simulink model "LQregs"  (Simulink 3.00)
settings: Solver=ode45  StartTime=0.0  StopTime=100  RelTol=1e-3

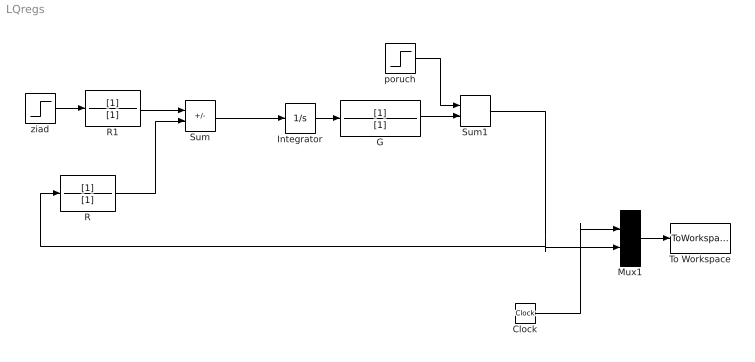
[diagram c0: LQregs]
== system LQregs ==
  Clock : Clock
  G : TransferFcn  Numerator=[1]  Denominator=[1]
  Integrator : Integrator  ExternalReset=none  InitialConditionSource=internal  InitialCondition=0  LimitOutput=off  UpperSaturationLimit=inf  LowerSaturationLimit=-inf  ShowSaturationPort=off  ShowStatePort=off  AbsoluteTolerance=auto
  Mux1 : Mux  Inputs=2
  R : TransferFcn  Numerator=[1]  Denominator=[1]
  R1 : TransferFcn  Numerator=[1]  Denominator=[1]
  Sum : Sum  Inputs=+-  SaturateOnIntegerOverflow=on
  Sum1 : Sum  Inputs=++  SaturateOnIntegerOverflow=on
  To Workspace : ToWorkspace  VariableName=simout  SampleTime=-1  SaveFormat=Matrix
  poruch : Step  Time=50  Before=0  After=2  SampleTime=0
  ziad : Step  Time=0  Before=0  After=5  SampleTime=0
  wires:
  Integrator/1 -> G/1
  G/1 -> Sum1/2
  poruch/1 -> Sum1/1
  ziad/1 -> R1/1
  R1/1 -> Sum/1
  R/1 -> Sum/2
  Sum/1 -> Integrator/1
  Mux1/1 -> To Workspace/1
  Sum1/1 -> R/1, Mux1/2
  Clock/1 -> Mux1/1
